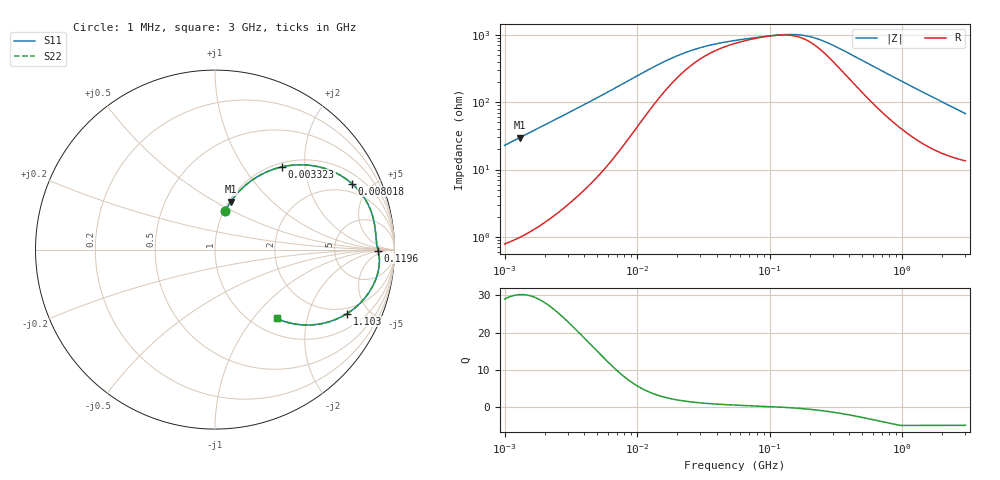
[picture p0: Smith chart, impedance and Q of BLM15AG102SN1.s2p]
! BLM15AG102SN1
# Hz S RI R 50
!Freq.(Hz) S11(Real) S11(Imag) S21(Real) S21(Imag) S12(Real) S12(Imag) S22(Real) S22(Imag)
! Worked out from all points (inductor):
!   401 points, 1 MHz to 3 GHz, reference 50 ohm
!   read as one part in series: L = 3.64 uH near 1.041 MHz
!   highest Q = 30.2 at 1.297 MHz (marker M1), where L = 3.64 uH
!   self-resonance near 110 MHz
!   S11 on the Smith chart (normalised r, x): 1 MHz: 1.02, +0.46; 3.323 MHz: 1.07, +1.53; 8.018 MHz: 1.48, +3.84; 119.6 MHz: 21, -1; 1.103 GHz: 1.68, -3.61; 3 GHz: 1.27, -1.33
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1000000  0.0563 0.214  0.9437 -0.214  0.9437 -0.214  0.0563 0.214
1297199  0.0883 0.2677  0.9117 -0.2677  0.9117 -0.2677  0.0883 0.2677
2097170  0.196 0.3793  0.804 -0.3793  0.804 -0.3793  0.196 0.3793
3323290  0.3748 0.4612  0.6252 -0.4612  0.6252 -0.4612  0.3748 0.4612
3823119  0.441 0.4712  0.559 -0.4712  0.559 -0.4712  0.441 0.4712
5372736  0.6053 0.454  0.3947 -0.454  0.3947 -0.454  0.6053 0.454
8017732  0.7626 0.368  0.2374 -0.368  0.2374 -0.368  0.7626 0.368
1.061086e7  0.8309 0.2897  0.1691 -0.2897  0.1691 -0.2897  0.8309 0.2897
1.461624e7  0.8714 0.2081  0.1286 -0.2081  0.1286 -0.2081  0.8714 0.2081
2.054061e7  0.8884 0.1421  0.1116 -0.1421  0.1116 -0.1421  0.8884 0.1421
2.773354e7  0.894 0.1006  0.106 -0.1006  0.106 -0.1006  0.894 0.1006
3.820236e7  0.8968 0.0686  0.1032 -0.0686  0.1032 -0.0686  0.8968 0.0686
5.477226e7  0.8993 0.042  0.1007 -0.042  0.1007 -0.042  0.8993 0.042
1.195584e8  0.9089 -0.00551  0.0911 0.00551  0.0911 0.00551  0.9089 -0.00551
1.614254e8  0.9135 -0.0283  0.0865 0.0283  0.0865 0.0283  0.9135 -0.0283
2.094008e8  0.916 -0.0534  0.084 0.0534  0.084 0.0534  0.916 -0.0534
2.827291e8  0.9147 -0.0902  0.0853 0.0902  0.0853 0.0902  0.9147 -0.0902
4.480278e8  0.896 -0.1649  0.104 0.1649  0.104 0.1649  0.896 -0.1649
8.005644e8  0.8186 -0.288  0.1814 0.288  0.1814 0.288  0.8186 -0.288
1.10276e9  0.7348 -0.3571  0.2652 0.3571  0.2652 0.3571  0.7348 -0.3571
1.818868e9  0.5444 -0.4191  0.4556 0.4191  0.4556 0.4191  0.5444 -0.4191
3e9  0.3429 -0.3838  0.6571 0.3838  0.6571 0.3838  0.3429 -0.3838
